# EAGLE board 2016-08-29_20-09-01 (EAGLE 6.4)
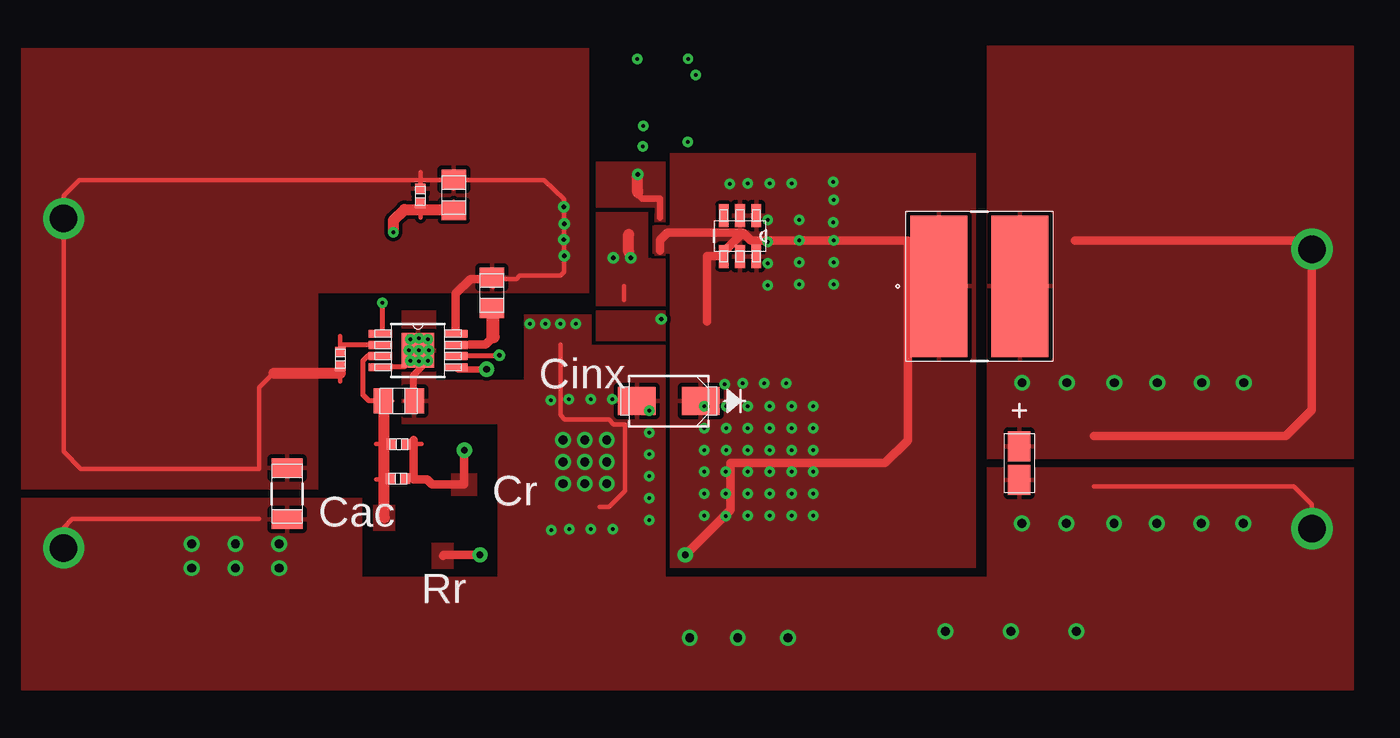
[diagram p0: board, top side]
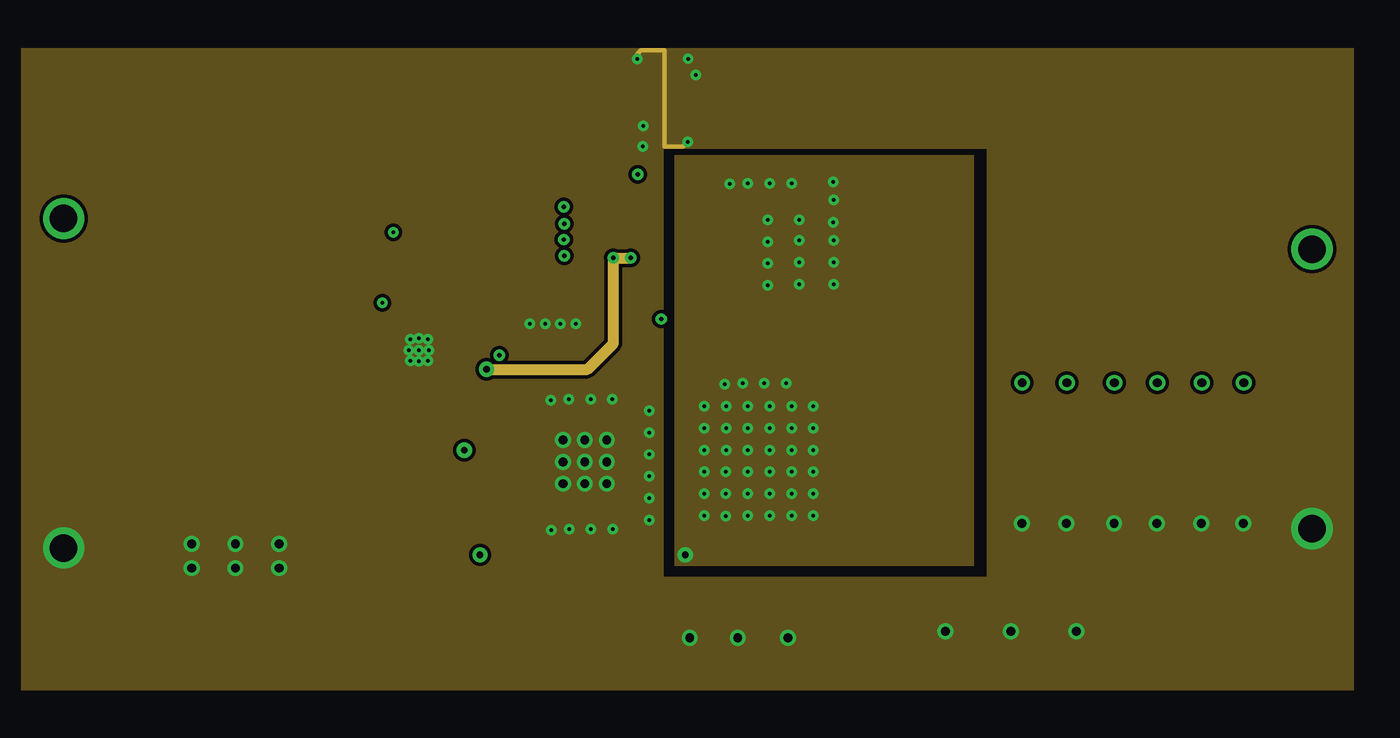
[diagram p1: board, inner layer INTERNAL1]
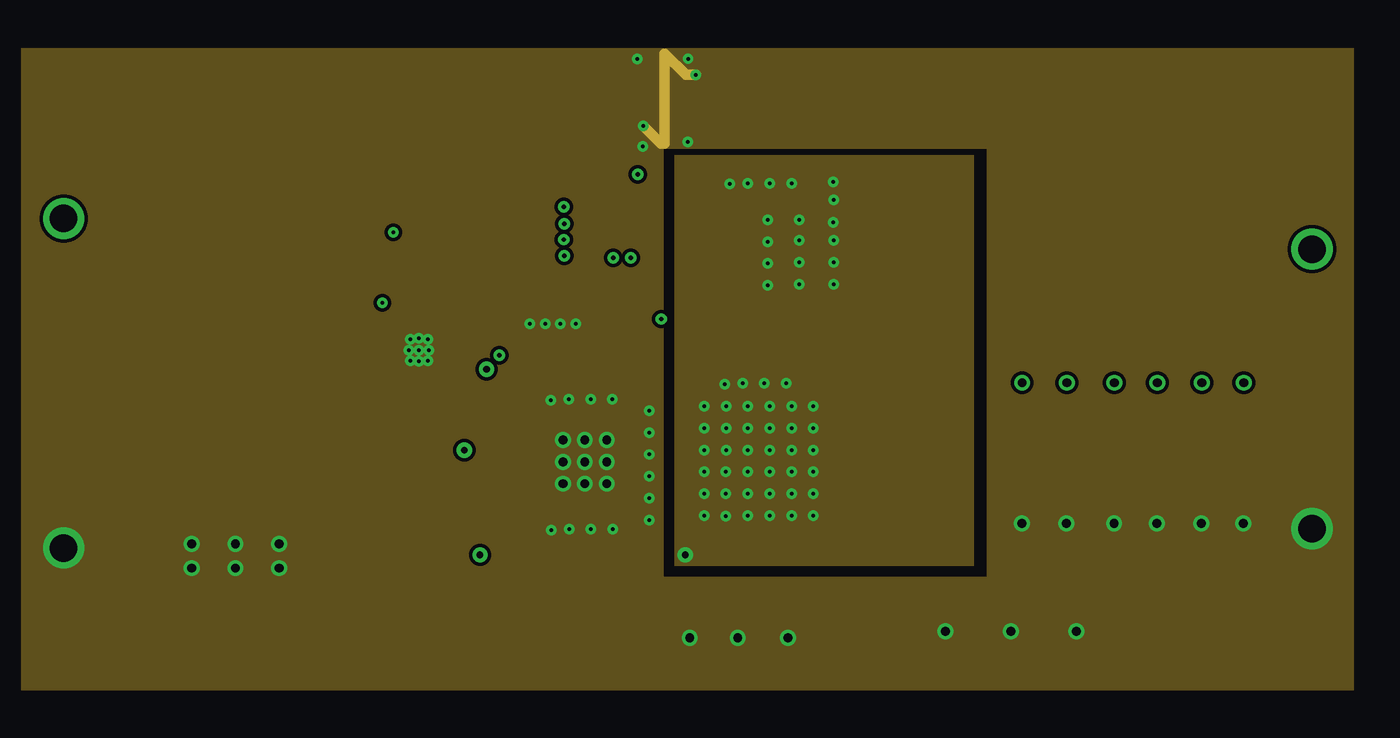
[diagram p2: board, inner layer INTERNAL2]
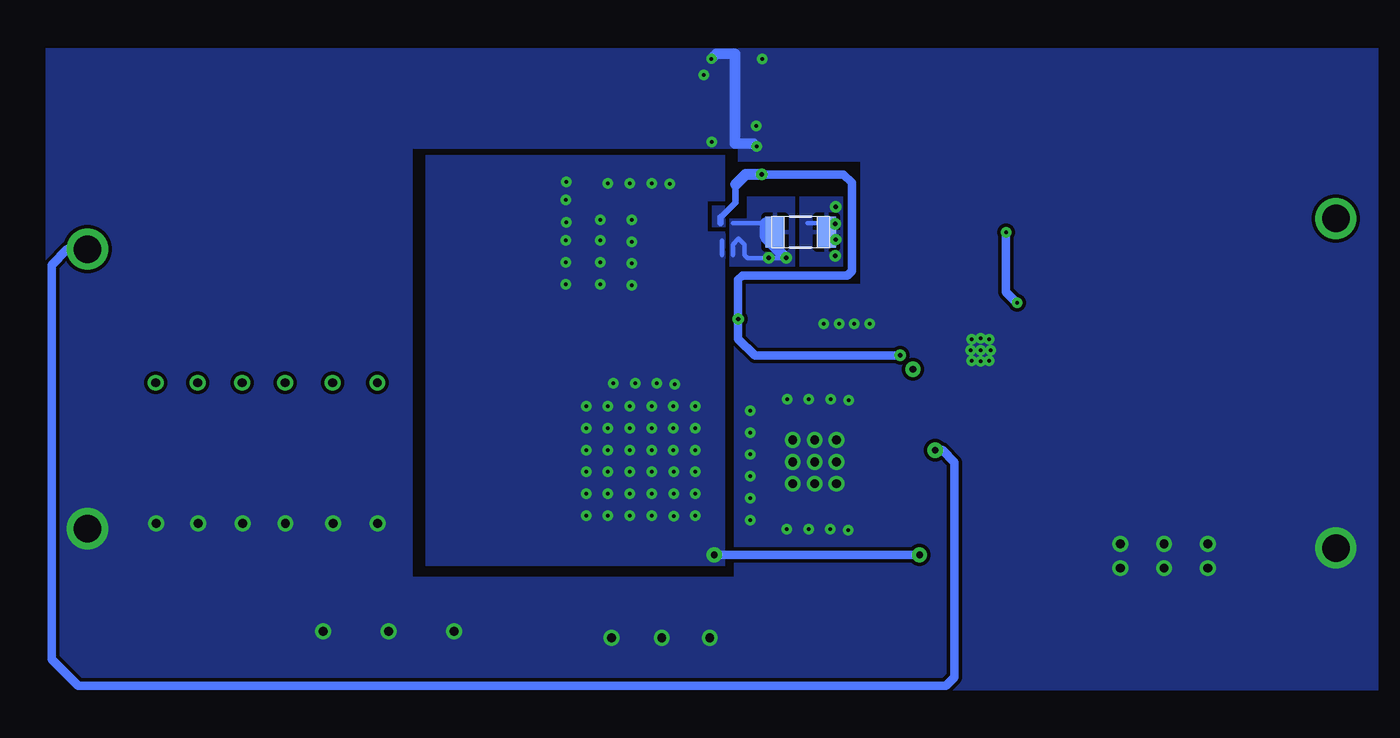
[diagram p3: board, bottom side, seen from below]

No outline drawn. Coordinates in mm, seen from the top.
Copper layers ((1*2)+(15*16)): TOP / INTERNAL1 / layer 15 / BOTTOM

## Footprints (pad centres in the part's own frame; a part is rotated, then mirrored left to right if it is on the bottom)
0805 = smd 1.118 x 1.448: 1 -0.902,0; 2 0.902,0
0402 = smd 0.559 x 0.61: 1 -0.419,0; 2 0.419,0
1206_190 = smd 1.118 x 1.803: 1 -1.499,0; 2 1.499,0
3216-18 = smd 1.753 x 1.295: 1 -0.978,0; 2 0.978,0
SMA = smd 2.184 x 1.626: 1 -1.854,0; 2 1.854,0
TP-1502 = drill 0.813 round: 1 0,0
VLP8040 = smd 3.302 x 8.204: 1 -2.349,0; 2 2.349,0
SOT-23-6 = smd 1.321 x 0.559: 1 -1.194,0.95; 2 -1.194,0; 3 -1.194,-0.95; 4 1.194,-0.95; 5 1.194,0; 6 1.194,0.95
1206 = smd 1.118 x 1.803: 1 -1.499,0; 2 1.499,0
MUY08A = smd 1.372 x 0.457: 1 -2.197,0.975; 2 -2.197,0.325; 3 -2.197,-0.325; 4 -2.197,-0.975; 5 2.197,-0.975; 6 2.197,-0.325; 7 2.197,0.325; 8 2.197,0.975 | smd 1.88 x 2.007: 9 0,0

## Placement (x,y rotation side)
Cadj  [0805]  50.8,54.58 270 top
Cff  [0402]  47.55,38.07 180 top
Cin  [1206_190]  41.1,37.21 270 top
Cout  [3216-18]  83.67,38.99 270 top
Cvcc  [0805]  53.01,48.9 270 top
D1  [SMA]  63.3,42.6 180 top
GND  [TP-1502]  100.63,35.13 0 top
GND1  [TP-1502]  28.09,34.04 0 top
L1  [VLP8040]  81.36,49.28 0 top
M1  [SOT-23-6]  67.44,52.2 270 top
Radj  [0402]  48.84,54.53 270 top
Rfb1  [0805]  47.6,42.6 0 top
Rfb2  [0402]  47.6,40.08 180 top
Rsns  [1206]  59.23,52.43 180 bottom
Rt  [0402]  44.2,45.06 90 top
U1  [MUY08A]  48.72,45.54 0 top
VIN  [TP-1502]  28.09,53.19 0 top
VOUT  [TP-1502]  100.63,51.44 0 top

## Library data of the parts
Cadj = ultra-librarian; RefDes: Cadj; Type: CL21C102JBCNFNC
Cff = ultra-librarian; RefDes: Cff; Type: GRM1555C1H431GA01D
Cin = ultra-librarian; RefDes: Cin; Type: GRM31CR71H225KA88L
Cout = ultra-librarian; RefDes: Cout; Type: TPSA336K006R0600
Cvcc = ultra-librarian; RefDes: Cvcc; Type: 0805YC474KAT2A
D1 = ultra-librarian; RefDes: D1; Type: B340A-13-F
GND = ultra-librarian; RefDes: GND; Type: TP-1502
GND1 = ultra-librarian; RefDes: GND1; Type: TP-1502
L1 = ultra-librarian; RefDes: L1; Type: VLP8040T-100M
M1 = ultra-librarian; RefDes: M1; Type: FDC5614P
Radj = ultra-librarian; RefDes: Radj; Type: CRCW04021K05FKED
Rfb1 = ultra-librarian; RefDes: Rfb1; Type: RT0805BRD076K12L
Rfb2 = ultra-librarian; RefDes: Rfb2; Type: CRCW040210K0FKED
Rsns = ultra-librarian; RefDes: Rsns; Type: CSR1206FK10L0
Rt = ultra-librarian; RefDes: Rt; Type: CRCW040229K4FKED
U1 = ultra-librarian; RefDes: U1; Type: LM25085MY/NOPB
VIN = ultra-librarian; RefDes: VIN; Type: TP-1502
VOUT = ultra-librarian; RefDes: VOUT; Type: TP-1502

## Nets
0: Cin.2 Cout.2 D1.2 GND1.1 GND.1 Rfb1.2 U1.4 U1.9
1: Cff.2 Rfb1.1 Rfb2.2 U1.3
2: Rt.2 U1.2
3: Cadj.1 Cin.1 Cvcc.1 Radj.1 Rsns.1 Rt.1 U1.8 VIN.1
4: M1.3 U1.6
5: M1.4 Rsns.2 U1.5
6: Cadj.2 Radj.2 U1.1
7: Cvcc.2 U1.7
8: D1.1 L1.1 M1.1 M1.2 M1.5 M1.6
9: Cff.1 Cout.1 L1.2 Rfb2.1 VOUT.1

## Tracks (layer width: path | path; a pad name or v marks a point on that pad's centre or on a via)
0  (via drill 0.2 pad 0.61, 0.51 pad 0.91, 1.6 pad 2.21)
  TOP 0.254: v100.69,35.18 100.69,36.6 99.62,37.64 88.01,37.64 | v28.12,34.06 28.12,35.23 28.63,35.74 39.5,35.74 | 59.26,36.45 59.82,36.45 60.1,36.7 60.76,37.36 60.76,41.25 60.1,41.25 59.82,41.53 59.26,41.53 57.25,41.53 57,41.78 57,45.9 | 47.98,42.61 48.92,42.61
  TOP 0.305: v48.26,44.93 47.93,44.6 46.63,44.6
  TOP 0.406: v49.28,44.93 48.46,44.12 48.46,42.62
  INTERNAL1 0.254: v64.39,57.66 64.14,57.4 63.04,57.4 63.04,62.99 61.67,62.99 61.47,62.79 v61.47,62.48
  INTERNAL2 0.61: v64.87,61.57 64.29,61.57 63.04,62.81 63.04,57.58 62.84,57.58 v61.82,58.6
  BOTTOM 0.61: v61.8,57.4 61.98,57.58 63.04,57.58 63.04,62.81 64.11,62.81 v64.41,62.51
  other vias: 62.15,42.04 62.15,40.77 62.15,39.5 62.15,38.23 62.15,36.96 62.15,35.69 60.02,42.7 58.75,42.7 57.48,42.7 56.44,42.65 60.05,35.15 58.78,35.15 57.51,35.15 56.46,35.1 48.77,44.91 48.77,46.25 48.18,45.57 49.35,45.57 86.41,35.48 96.7,35.48 94.26,35.48 59.69,40.34 59.69,39.07 59.69,37.8 58.42,37.8 57.15,37.8 58.42,40.34 57.15,40.34 57.15,39.07 58.42,39.07 89.18,35.48 91.67,35.48 48.77,45.57 49.28,46.2 48.26,46.2 55.22,47.09 57,47.09 56.11,47.09 57.89,47.09 83.82,35.48 87,29.21 83.19,29.21 79.38,29.21 67.31,28.83 70.23,28.83 64.52,28.83 40.64,34.29 35.56,32.89 40.64,32.89 38.1,34.29 38.1,32.89 35.56,34.29
  pour TOP (rank 6): 25.65,36.96 45.47,36.96 45.47,32.38 53.34,32.38 53.34,41.27 47.75,41.27 47.75,47.88 49.78,47.88 49.78,43.81 54.89,43.81 54.89,47.62 58.8,47.62 58.8,45.85 63.12,45.85 63.12,32.38 81.79,32.38 81.79,38.73 103.12,38.73 103.12,25.78 25.65,25.78
  pour BOTTOM (rank 6): 25.65,63.12 62.87,63.12 62.87,56.52 55.75,56.52 55.75,49.4 63.12,49.4 63.12,32.38 81.79,32.38 81.79,57.28 63.12,57.28 63.12,63.12 103.12,63.12 103.12,25.78 25.65,25.78
  pour INTERNAL1 (rank 6): 25.65,63.12 62.99,63.12 62.99,32.38 81.79,32.38 81.79,57.28 63.12,57.28 63.12,63.12 103.12,63.12 103.12,25.78 25.65,25.78
  pour INTERNAL2: 25.65,63.12 62.99,63.12 62.99,32.38 81.79,32.38 81.79,57.28 63.12,57.28 63.12,63.12 103.12,63.12 103.12,25.78 25.65,25.78
1
  TOP 0.254: 46.28,38.04 47.22,38.04 | 46.28,42.61 47.22,42.61 | 46.28,40.12 47.22,40.12
  TOP 0.305: 46.76,42.62 45.85,42.62 45.52,42.95 45.52,44.96 45.82,45.26 46.63,45.26
  TOP 0.635: 46.76,35.81 46.76,38.05 46.76,42.62
  pour TOP (rank 3): 46.1,35.05 46.1,36.55 47.4,36.55 47.4,35.05
2
  TOP 0.254: 44.2,45.92 44.2,45.9 | 44.18,45.44 44.18,46.38
  TOP 0.305: 44.2,45.9 46.63,45.9
3  (via drill 0.25 pad 0.61, 1.6 pad 2.21)
  TOP 0.254: 40.34,44.22 39.5,43.38 39.5,38.66 29.11,38.66 28.12,39.67 v28.12,53.21 28.12,54.53 29.03,55.45 48.9,55.45 56.06,55.45 57.2,54.33 57.2,50.09 57,49.89 54.63,49.89 54.46,49.71 53.09,49.71 | 48.88,54.97 48.88,55.91 | 53.07,49.23 53.07,50.16 | 44.18,43.74 44.18,44.68 | 50.79,54.97 50.79,55.91
  TOP 0.508: 50.9,46.74 50.9,48.84 51.77,49.71 53.09,49.71
  TOP 0.635: 40.34,44.22 44.2,44.22
  BOTTOM 0.254: 57.89,52.96 58.83,52.96
  other vias: 57.23,51.05 57.2,51.99 57.23,52.91 57.2,53.9
  pour TOP (rank 2): 55.3,49.1 55.3,50.67 58.67,50.67 58.67,49.1
  pour TOP (rank 4): 25.65,63.12 58.67,63.12 58.67,48.9 42.93,48.9 42.93,37.47 25.65,37.47
  pour BOTTOM (rank 5): 56.77,50.42 59.31,50.42 59.31,54.48 56.77,54.48
4  (via drill 0.25 pad 0.61)
  TOP 0.305: 50.9,45.26 v53.44,45.26
  TOP 0.381: 62.79,53.26 62.79,54.38 62.13,54.38 62.15,54.38 61.75,54.38 61.54,54.59 61.49,54.59 v61.49,55.78
  TOP 0.635: 61.49,54.74 v61.49,55.78 61.49,54.86
  BOTTOM 0.381: 63.88,52.96 63.88,53.29 | 63.86,53.29 63.02,54.13 63.02,55.19
  BOTTOM 0.508: v61.49,55.78 56.74,55.78 56.26,55.3 56.26,50.16 56.52,49.91 62.61,49.91 62.87,49.66 62.87,46.2 61.9,45.26 v53.44,45.26
  BOTTOM 0.635: 63.02,55.19 62.43,55.78 v61.49,55.78
  other vias: 62.87,47.37
  pour TOP: 62.46,53.01 62.46,53.49 63.12,53.49 63.12,53.01
  pour TOP (rank 4): 59.05,56.52 59.05,53.85 62.48,53.85 62.48,53.09 63.12,53.09 63.12,56.52
  pour TOP (rank 5): 59.05,47.88 59.05,46.1 63.12,46.1 63.12,47.88
  pour BOTTOM (rank 3): 63.6,52.73 63.6,53.19 63.98,53.19 63.98,52.73
  pour BOTTOM (rank 5): 63.63,53.98 64.39,53.98 64.39,52.7 63.63,52.7
5  (via drill 0.25 pad 0.61, 0.38 pad 0.89)
  TOP 0.254: 60.71,48.49 60.71,49.28
  TOP 0.381: 50.9,44.6 51.05,44.45 v52.7,44.45
  TOP 0.635: 60.96,51.28 60.96,52.3
  INTERNAL1 0.635: v61.09,50.93 v60.07,50.93 60.07,45.95 58.57,44.45 v52.7,44.45
  BOTTOM 0.254: v60.07,50.93 v61.09,50.93 62.33,50.93 62.51,51.1 62.51,51.71 62.84,52.05 63.17,51.71 63.17,51.1 | 61.27,52.96 | 61.27,52.96 62.51,52.96 63.17,52.96 | 60.78,52.96 61.72,52.96
  BOTTOM 0.635: v60.07,50.93 61.27,52.12 61.27,52.96
  pour TOP: 59.99,50.95 59.99,53.59 61.95,53.59 61.95,50.95
  pour TOP: 60.02,49.3 60.02,50.88 63.07,50.88 63.07,49.3
  pour TOP (rank 4): 59.05,53.59 62.1,53.59 62.1,50.93 63.12,50.93 63.12,48.13 59.05,48.13
  pour BOTTOM (rank 5): 63.37,50.42 63.37,53.21 62.36,53.21 62.36,54.48 59.56,54.48 59.56,50.42
6  (via drill 0.2 pad 0.61)
  TOP 0.254: 48.88,53.26 48.88,54.2 | 50.79,53.26 50.79,54.2
  TOP 0.305: 46.66,46.56 v46.66,48.31
  TOP 0.635: 50.8,53.75 48.9,53.75 47.93,53.75 47.3,53.11 v47.3,52.43
  BOTTOM 0.508: v46.66,48.31 47.3,48.95 v47.3,52.43
7
  TOP 0.254: 53.07,47.52 53.07,48.46
  TOP 0.406: 50.9,45.9 51.71,45.9
  TOP 0.508: 53.09,46.33 52.65,45.9 51.71,45.9
  TOP 0.762: 53.09,46.33 53.09,48.01
8  (via drill 0.2 pad 0.61, 0.38 pad 0.89)
  TOP 0.508: 67.61,52.4 68.07,51.94 77.19,51.94 77.19,40.31 75.87,38.99 69.47,38.99 66.88,38.99 | 67.61,52.4 66.24,51.03 65.51,51.03 65.51,49.76 65.51,48.49 65.51,47.22 | 67.61,52.4 63.22,52.4 62.79,51.97 62.79,51.36 | 66.88,38.94 66.88,36.27 v64.26,33.66 | v52.32,33.66 50.22,33.66 50.16,33.6
  BOTTOM 0.254: 63.8,51.1 63.8,51.94
  BOTTOM 0.508: v52.32,33.66 v64.26,33.66
  other vias: 69.04,51.87 70.87,51.94 72.9,51.94 72.85,52.98 72.9,50.67 70.87,50.67 72.9,54.31 72.85,55.35 70.43,55.27 69.16,55.27 67.89,55.27 66.85,55.22 70.13,43.64 68.86,43.64 67.59,43.64 66.55,43.59 70.87,53.14 66.6,35.92 66.6,38.48 66.6,37.21 65.35,37.21 65.35,35.94 69.04,49.33 69.04,50.6 69.04,53.14 67.89,35.94 69.16,35.94 70.43,35.94 65.35,38.48 65.35,39.75 65.35,41.02 65.35,42.29 66.62,42.29 66.62,41.02 66.62,39.75 67.89,42.29 69.16,42.29 67.89,41.02 69.16,41.02 67.89,39.75 69.16,39.75 67.89,38.48 69.16,38.48 67.89,37.21 69.16,37.21 70.43,42.29 70.43,41.02 70.43,39.75 70.43,38.48 70.43,37.21 71.7,35.94 71.7,37.21 71.7,38.48 71.7,39.75 71.7,41.02 71.7,42.29 70.87,49.4 72.9,49.4
  pour TOP: 62.46,51.05 62.46,51.54 63.12,51.54 63.12,51.05
  pour TOP: 62.46,52.35 62.46,52.83 63.12,52.83 63.12,52.35
  pour TOP (rank 2): 49.5,32.84 49.5,34.34 50.8,34.34 50.8,32.84
  pour TOP (rank 4): 81.15,57.02 81.15,32.89 63.37,32.89 63.37,51.18 62.36,51.18 62.36,52.83 63.37,52.83 63.37,57.02
  pour BOTTOM (rank 3): 63.6,50.88 63.6,51.33 63.98,51.33 63.98,50.88
  pour BOTTOM (rank 3): 63.6,51.51 63.6,52.35 63.98,52.35 63.98,51.51
  pour BOTTOM (rank 5): 81.03,56.9 81.03,33.02 63.63,33.02 63.63,52.45 64.64,52.45 64.64,54.23 63.63,54.23 63.63,56.9
  pour INTERNAL1 (rank 6): 63.63,33.02 63.63,56.9 81.03,56.9 81.03,33.02
  pour INTERNAL2 (rank 6): 63.63,33.02 63.63,56.9 81.03,56.9 81.03,33.02
9  (via drill 0.38 pad 0.89, 0.51 pad 0.91, 1.6 pad 2.21)
  TOP 0.254: 47.98,38.04 48.92,38.04 | 47.98,40.12 48.92,40.12
  TOP 0.508: v51.41,39.75 51.41,37.74 49.53,37.74 49.25,38.05 48.46,38.05 48.46,40.34 | 88.01,40.56 99.16,40.56 100.69,42.09 v100.69,51.44 100.18,51.94 86.89,51.94
  BOTTOM 0.508: v51.41,39.75 50.98,39.75 50.29,39.04 50.29,26.54 50.8,26.04 101.22,26.04 102.77,27.58 102.77,50.52 101.85,51.44 v100.69,51.44
  other vias: 83.85,43.66 91.69,43.66 89.2,43.66 94.28,43.66 96.72,43.66 86.44,43.66
  pour TOP (rank 2): 50.65,37.08 50.65,38.38 52.15,38.38 52.15,37.08
  pour TOP (rank 4): 103.12,63.27 103.12,39.24 81.79,39.24 81.79,63.27

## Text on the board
ASSYNOTES: Cinx | Cr | Cac | Rr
